| / 7\'7   Xilinx XC1700E I/O Buffer IBIS File
| \ \   Xilinx Inc.
| / /   2100 Logic Drive
| \_\/.\   San Jose,   CA 95124
[IBIS ver]   2.1
[File name]   xc1700e.ibs
[File Rev]   1.0
[Date]   Feb. 10, 2000
[Source]   Spice netlist
[Notes]   - Best/worse process data included in the model
   - Created by Joey Jia x4437
[Disclaimer] The data in this model is derived from SPICE simulations
   using modeling information extracted from the target pro-
   cess. While a great deal of care has been take to provide
   information that is accurate, this model is considered
   preliminary as it has not been verified by actual silicon
   measurement. Treat the data in this model as preliminary
   until actual silicon verification is performed.
[Copyright]   Xilinx Inc. All right reserved
|   Component XC1736E_PD8
[Component]   XC1736E_PD8
[Manufacturer]   Xilinx Inc.
[Package]
| variable   typ   min   max
R_pkg   89.00m   80.000m   98.00m
L_pkg   5.850nH   4.200nH   7.500nH
C_pkg   0.950pF   0.700pF   1.200pF
[Pin]  signal_name   model_name   R_pin   L_pin   C_pin
io   datap   IO_1700E   NA   NA   NA
| End [Component] XC1736E_PD8
|   Component XC1736E_SO8
[Component]   XC1736E_SO8
[Manufacturer]   Xilinx Inc.
[Package]
| variable   typ   min   max
R_pkg   42.50m   41.000m   44.00m
L_pkg   1.800nH   1.600nH   2.000nH
C_pkg   0.300pF   0.300pF   0.300pF
[Pin]  signal_name   model_name   R_pin   L_pin   C_pin
io   datap   IO_1700E   NA   NA   NA
| End [Component] XC1736E_SO8
|   Component XC1736E_VO8
[Component]   XC1736E_VO8
[Manufacturer]   Xilinx Inc.
[Package]
| variable   typ   min   max
R_pkg   42.50m   41.000m   44.00m
L_pkg   1.800nH   1.600nH   2.000nH
C_pkg   0.300pF   0.300pF   0.300pF
[Pin]  signal_name   model_name   R_pin   L_pin   C_pin
io   datap   IO_1700E   NA   NA   NA
| End [Component] XC1736E_VO8
|   Component XC1736E_PC20
[Component]   XC1736E_PC20
[Manufacturer]   Xilinx Inc.
[Package]
| variable   typ   min   max
R_pkg   56.50m   53.000m   60.00m
L_pkg   3.300nH   3.000nH   3.600nH
C_pkg   0.700pF   0.700pF   0.700pF
[Pin]  signal_name   model_name   R_pin   L_pin   C_pin
io   datap   IO_1700E   NA   NA   NA
| End [Component] XC1736E_PC20
|   Component XC1765E_PD8
[Component]   XC1765E_PD8
[Manufacturer]   Xilinx Inc.
[Package]
| variable   typ   min   max
R_pkg   89.00m   80.000m   98.00m
L_pkg   5.850nH   4.200nH   7.500nH
C_pkg   0.950pF   0.700pF   1.200pF
[Pin]  signal_name   model_name   R_pin   L_pin   C_pin
io   datap   IO_1700E   NA   NA   NA
| End [Component] XC1765E_PD8
|   Component XC1765E_SO8
[Component]   XC1765E_SO8
[Manufacturer]   Xilinx Inc.
[Package]
| variable   typ   min   max
R_pkg   42.50m   41.000m   44.00m
L_pkg   1.800nH   1.600nH   2.000nH
C_pkg   0.300pF   0.300pF   0.300pF
[Pin]  signal_name   model_name   R_pin   L_pin   C_pin
io   datap   IO_1700E   NA   NA   NA
| End [Component] XC1765E_SO8
|   Component XC1765E_VO8
[Component]   XC1765E_VO8
[Manufacturer]   Xilinx Inc.
[Package]
| variable   typ   min   max
R_pkg   42.50m   41.000m   44.00m
L_pkg   1.800nH   1.600nH   2.000nH
C_pkg   0.300pF   0.300pF   0.300pF
[Pin]  signal_name   model_name   R_pin   L_pin   C_pin
io   datap   IO_1700E   NA   NA   NA
| End [Component] XC1765E_VO8
|   Component XC1765E_PC20
[Component]   XC1765E_PC20
[Manufacturer]   Xilinx Inc.
[Package]
| variable   typ   min   max
R_pkg   56.50m   53.000m   60.00m
L_pkg   3.300nH   3.000nH   3.600nH
C_pkg   0.700pF   0.700pF   0.700pF
[Pin]  signal_name   model_name   R_pin   L_pin   C_pin
io   datap   IO_1700E   NA   NA   NA
| End [Component] XC1765E_PC20
|   Component XC17128E_PD8
[Component]   XC17128E_PD8
[Manufacturer]   Xilinx Inc.
[Package]
| variable   typ   min   max
R_pkg   89.00m   80.000m   98.00m
L_pkg   5.850nH   4.200nH   7.500nH
C_pkg   0.950pF   0.700pF   1.200pF
[Pin]  signal_name   model_name   R_pin   L_pin   C_pin
io   datap   IO_1700E   NA   NA   NA
| End [Component] XC17128E_PD8
|   Component XC17128E_VO8
[Component]   XC17128E_VO8
[Manufacturer]   Xilinx Inc.
[Package]
| variable   typ   min   max
R_pkg   42.50m   41.000m   44.00m
L_pkg   1.800nH   1.600nH   2.000nH
C_pkg   0.300pF   0.300pF   0.300pF
[Pin]  signal_name   model_name   R_pin   L_pin   C_pin
io   datap   IO_1700E   NA   NA   NA
| End [Component] XC17128E_VO8
|   Component XC17128E_PC20
[Component]   XC17128E_PC20
[Manufacturer]   Xilinx Inc.
[Package]
| variable   typ   min   max
R_pkg   56.50m   53.000m   60.00m
L_pkg   3.300nH   3.000nH   3.600nH
C_pkg   0.700pF   0.700pF   0.700pF
[Pin]  signal_name   model_name   R_pin   L_pin   C_pin
io   datap   IO_1700E   NA   NA   NA
| End [Component] XC17128E_PC20
|   Component XC17256E_PD8
[Component]   XC17256E_PD8
[Manufacturer]   Xilinx Inc.
[Package]
| variable   typ   min   max
R_pkg   89.00m   80.000m   98.00m
L_pkg   5.850nH   4.200nH   7.500nH
C_pkg   0.950pF   0.700pF   1.200pF
[Pin]  signal_name   model_name   R_pin   L_pin   C_pin
io   datap   IO_1700E   NA   NA   NA
| End [Component] XC17256E_PD8
|   Component XC17256E_VO8
[Component]   XC17256E_VO8
[Manufacturer]   Xilinx Inc.
[Package]
| variable   typ   min   max
R_pkg   42.50m   41.000m   44.00m
L_pkg   1.800nH   1.600nH   2.000nH
C_pkg   0.300pF   0.300pF   0.300pF
[Pin]  signal_name   model_name   R_pin   L_pin   C_pin
io   datap   IO_1700E   NA   NA   NA
| End [Component] XC17256E_VO8
|   Component XC17256E_PC20
[Component]   XC17256E_PC20
[Manufacturer]   Xilinx Inc.
[Package]
| variable   typ   min   max
R_pkg   56.50m   53.000m   60.00m
L_pkg   3.300nH   3.000nH   3.600nH
C_pkg   0.700pF   0.700pF   0.700pF
[Pin]  signal_name   model_name   R_pin   L_pin   C_pin
io   datap   IO_1700E   NA   NA   NA
| End [Component] XC17256E_PC20
|   Component XC1765EL_PD8
[Component]   XC1765EL_PD8
[Manufacturer]   Xilinx Inc.
[Package]
| variable   typ   min   max
R_pkg   89.00m   80.000m   98.00m
L_pkg   5.850nH   4.200nH   7.500nH
C_pkg   0.950pF   0.700pF   1.200pF
[Pin]  signal_name   model_name   R_pin   L_pin   C_pin
io   datap   IO_1700EL   NA   NA   NA
| End [Component] XC1765EL_PD8
|   Component XC1765EL_SO8
[Component]   XC1765EL_SO8
[Manufacturer]   Xilinx Inc.
[Package]
| variable   typ   min   max
R_pkg   42.50m   41.000m   44.00m
L_pkg   1.800nH   1.600nH   2.000nH
C_pkg   0.300pF   0.300pF   0.300pF
[Pin]  signal_name   model_name   R_pin   L_pin   C_pin
io   datap   IO_1700EL   NA   NA   NA
| End [Component] XC1765EL_SO8
|   Component XC1765EL_VO8
[Component]   XC1765EL_VO8
[Manufacturer]   Xilinx Inc.
[Package]
| variable   typ   min   max
R_pkg   42.50m   41.000m   44.00m
L_pkg   1.800nH   1.600nH   2.000nH
C_pkg   0.300pF   0.300pF   0.300pF
[Pin]  signal_name   model_name   R_pin   L_pin   C_pin
io   datap   IO_1700EL   NA   NA   NA
| End [Component] XC1765EL_VO8
|   Component XC1765EL_PC20
[Component]   XC1765EL_PC20
[Manufacturer]   Xilinx Inc.
[Package]
| variable   typ   min   max
R_pkg   56.50m   53.000m   60.00m
L_pkg   3.300nH   3.000nH   3.600nH
C_pkg   0.700pF   0.700pF   0.700pF
[Pin]  signal_name   model_name   R_pin   L_pin   C_pin
io   datap   IO_1700EL   NA   NA   NA
| End [Component] XC1765EL_PC20
|   Component XC17128EL_PD8
[Component]   XC17128EL_PD8
[Manufacturer]   Xilinx Inc.
[Package]
| variable   typ   min   max
R_pkg   89.00m   80.000m   98.00m
L_pkg   5.850nH   4.200nH   7.500nH
C_pkg   0.950pF   0.700pF   1.200pF
[Pin]  signal_name   model_name   R_pin   L_pin   C_pin
io   datap   IO_1700EL   NA   NA   NA
| End [Component] XC17128EL_PD8
|   Component XC17128EL_VO8
[Component]   XC17128EL_VO8
[Manufacturer]   Xilinx Inc.
[Package]
| variable   typ   min   max
R_pkg   42.50m   41.000m   44.00m
L_pkg   1.800nH   1.600nH   2.000nH
C_pkg   0.300pF   0.300pF   0.300pF
[Pin]  signal_name   model_name   R_pin   L_pin   C_pin
io   datap   IO_1700EL   NA   NA   NA
| End [Component] XC17128EL_VO8
|   Component XC17128EL_PC20
[Component]   XC17128EL_PC20
[Manufacturer]   Xilinx Inc.
[Package]
| variable   typ   min   max
R_pkg   56.50m   53.000m   60.00m
L_pkg   3.300nH   3.000nH   3.600nH
C_pkg   0.700pF   0.700pF   0.700pF
[Pin]  signal_name   model_name   R_pin   L_pin   C_pin
io   datap   IO_1700EL   NA   NA   NA
| End [Component] XC17128EL_PC20
|   Component XC17256EL_PD8
[Component]   XC17256EL_PD8
[Manufacturer]   Xilinx Inc.
[Package]
| variable   typ   min   max
R_pkg   89.00m   80.000m   98.00m
L_pkg   5.850nH   4.200nH   7.500nH
C_pkg   0.950pF   0.700pF   1.200pF
[Pin]  signal_name   model_name   R_pin   L_pin   C_pin
io   datap   IO_1700EL   NA   NA   NA
| End [Component] XC17256EL_PD8
|   Component XC17256EL_VO8
[Component]   XC17256EL_VO8
[Manufacturer]   Xilinx Inc.
[Package]
| variable   typ   min   max
R_pkg   42.50m   41.000m   44.00m
L_pkg   1.800nH   1.600nH   2.000nH
C_pkg   0.300pF   0.300pF   0.300pF
[Pin]  signal_name   model_name   R_pin   L_pin   C_pin
io   datap   IO_1700EL   NA   NA   NA
| End [Component] XC17256EL_VO8
|   Component XC17256EL_PC20
[Component]   XC17256EL_PC20
[Manufacturer]   Xilinx Inc.
[Package]
| variable   typ   min   max
R_pkg   56.50m   53.000m   60.00m
L_pkg   3.300nH   3.000nH   3.600nH
C_pkg   0.700pF   0.700pF   0.700pF
[Pin]  signal_name   model_name   R_pin   L_pin   C_pin
io   datap   IO_1700EL   NA   NA   NA
| End [Component] XC17256EL_PC20
| Models and submodels in the file (2): IO_1700E (I/O), IO_1700EL (I/O)
